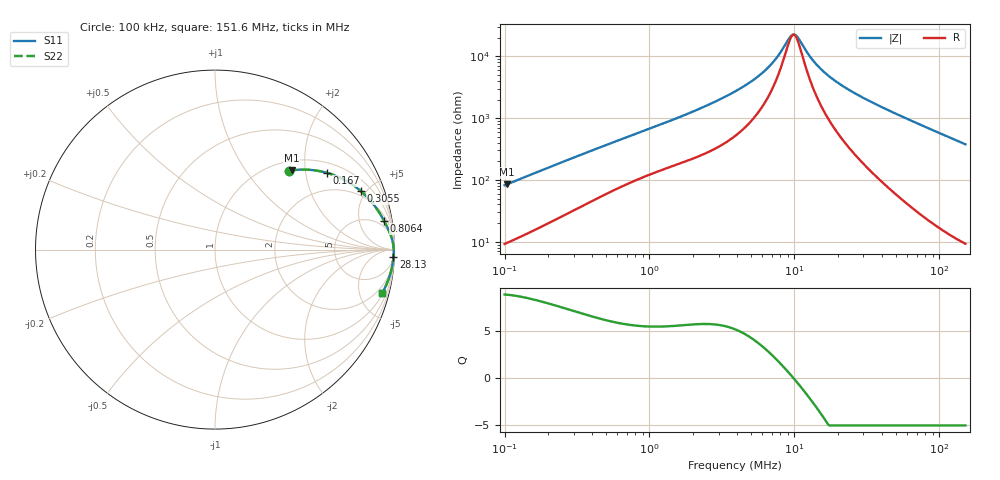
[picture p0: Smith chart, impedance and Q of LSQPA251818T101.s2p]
! LSQPA251818T101  S-PARAMETER MODEL  ( General Type )
! Model Generated by TAIYO YUDEN Corporation (http://www.ty-top.com)
! Version 3.0
! TAIYO YUDEN Control No. 160907NF25SB-FAC
! Copyright(c) 2007 TAIYO YUDEN CO.,LTD. All Rights Reserved.
! Product Description (link to TY-COMPAS)
! https://ds.yuden.co.jp/TYCOMPAS/or/detail?pn=LSQPA251818T101K&u=M
! Products Name : Inductors
! Characteristics :
!  Inductance : 100 uH , SRF(min) : 9.0 MHz , DC Resistance(max) : 4.81 Ohm
!  Rated Current : Saturation :160 mA , Temp Rise : 170 mA (40 degC)
!  Case Size : 2.5 x 1.8 / 0.098 x 0.071 [mm/inch] , Thickness : 1.8 / 0.071 [mm/inch]
!  (Conditions: Temperature = 25 degC , DC Bias Current/Voltage = 0A / 0V)
! External Node Assignments :
!  1  o---GGG---o  2
! GND o---------o GND
! Frequency Range : 0.1MHz  -  151.640846MHz  [ 402 STEP ]
# MHz S RI R 50
! Freq[MHz].  S11 Real  S11 Imag  S21 Real  S21 Imag  S12 Real  S12 Imag  S22 Real  S22 Imag
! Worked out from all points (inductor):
!   401 points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, 100 kHz to 151.6 MHz, reference 50 ohm
!   read as one part in series: L = 128 uH near 103.7 kHz
!   highest Q = 8.83 at 103.7 kHz (marker M1), where L = 129 uH
!   self-resonance near 9.728 MHz
!   S11 on the Smith chart (normalised r, x): 100 kHz: 1.18, +1.63; 167 kHz: 1.32, +2.65; 305.5 kHz: 1.66, +4.63; 806.4 kHz: 3, +11; 28.13 MHz: 5, -46; 151.6 MHz: 1.19, -7.55
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0.1  0.4112 0.4388  0.5888 -0.4388  0.5888 -0.4388  0.4112 0.4388
0.10373  0.4266 0.4412  0.5734 -0.4412  0.5734 -0.4412  0.4266 0.4412
0.166977  0.6255 0.4271  0.3745 -0.4271  0.3745 -0.4271  0.6255 0.4271
0.305544  0.8139 0.3249  0.1861 -0.3249  0.1861 -0.3249  0.8139 0.3249
0.341025  0.8374 0.3032  0.1626 -0.3032  0.1626 -0.3032  0.8374 0.3032
0.806367  0.9418 0.1608  0.0582 -0.1608  0.0582 -0.1608  0.9418 0.1608
1.162983  0.9623 0.1198  0.0377 -0.1198  0.0377 -0.1198  0.9623 0.1198
2.33212  0.9845 0.064  0.0155 -0.064  0.0155 -0.064  0.9845 0.064
3.894109  0.9917 0.0358  0.00826 -0.0358  0.00826 -0.0358  0.9917 0.0358
5.219642  0.9938 0.023  0.0062 -0.023  0.0062 -0.023  0.9938 0.023
6.502273  0.9947 0.0146  0.00526 -0.0146  0.00526 -0.0146  0.9947 0.0146
7.528034  0.9952 0.00937  0.00485 -0.00937  0.00485 -0.00937  0.9952 0.00937
9.20776  0.9955 0.0024  0.00448 -0.0024  0.00448 -0.0024  0.9955 0.0024
9.727699  0.9956 0.000524  0.00441 -0.000524  0.00441 -0.000524  0.9956 0.000524
10.46691  0.9957 -0.00198  0.00434 0.00198  0.00434 0.00198  0.9957 -0.00198
13.2799  0.9957 -0.0103  0.00428 0.0103  0.00428 0.0103  0.9957 -0.0103
15.0959  0.9957 -0.015  0.00434 0.015  0.00434 0.015  0.9957 -0.015
17.80031  0.9955 -0.0214  0.00452 0.0214  0.00452 0.0214  0.9955 -0.0214
28.1338  0.9941 -0.0428  0.00586 0.0428  0.00586 0.0428  0.9941 -0.0428
45.28783  0.9903 -0.0745  0.00973 0.0745  0.00973 0.0745  0.9903 -0.0745
84.40164  0.9748 -0.1415  0.0252 0.1415  0.0252 0.1415  0.9748 -0.1415
151.6408  0.9293 -0.2443  0.0707 0.2443  0.0707 0.2443  0.9293 -0.2443
